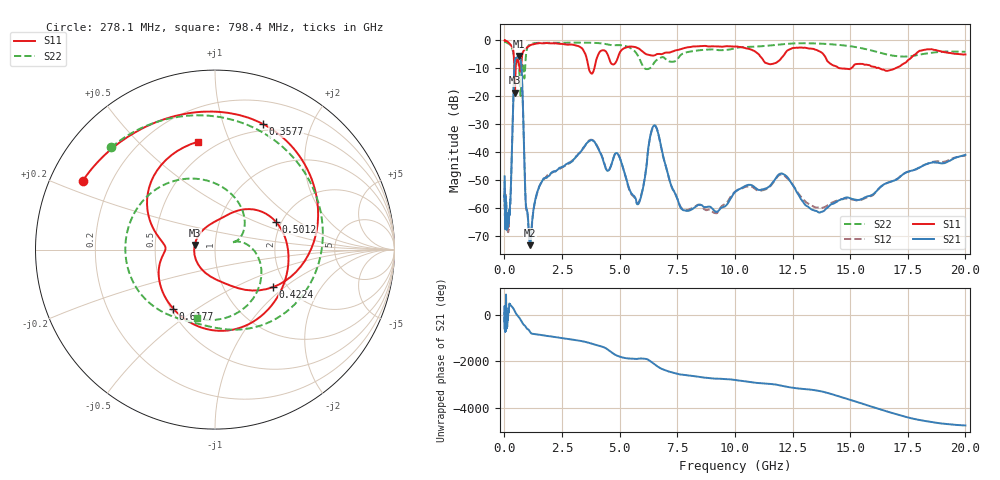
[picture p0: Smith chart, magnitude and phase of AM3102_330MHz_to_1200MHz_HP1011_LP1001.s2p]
! Date/Time: Tue, Sep 11, 2018 5:20 PM
! Network Analyzer: Agilent Technologies E8362B Rev: A.07.50.63
! Sweep from 0.010 to 20.000 GHz, 1601 Points, Sweep Type: LOG
! Power Supply: 4.949 V, 0.001 A
# Hz S DB R 50
!freq MagS11 AngS11 MagS21 AngS21 MagS12 AngS12 MagS22 AngS22
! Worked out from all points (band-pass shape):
!   1601 points, 10 MHz to 20 GHz, reference 50 ohm
!   highest |S21| = -5.53 dB at 638.6 MHz (marker M1); lowest = -73.4 dB at 1.113 GHz (marker M2)
!   |S21| within 3 dB of the highest: 440.3 MHz to 728.7 MHz (288.4 MHz wide, 49.3 % of centre)
!   lowest |S11| = -18.7 dB at 455.8 MHz (marker M3), VSWR 1.26, Z = 39.8 + j2.04 ohm
!   |S11| at or under -10 dB: 3.662 GHz to 3.902 GHz (240.6 MHz wide, 6.36 % of centre); 14.62 GHz to 15.03 GHz (408.4 MHz wide, 2.75 % of centre); 16.29 GHz to 16.95 GHz (666.5 MHz wide, 4.01 % of centre)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
!   |S22| runs from -19.8 to -0.2 dB; largest |S21 - S12| = 0.0096
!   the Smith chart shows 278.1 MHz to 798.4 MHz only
!   S11 on the Smith chart (normalised r, x): 278.1 MHz: 0.10, +0.24; 357.7 MHz: 0.43, +1.36; 422.4 MHz: 1.69, -0.83; 501.2 MHz: 1.87, +0.67; 617.7 MHz: 0.51, -0.40; 798.4 MHz: 0.40, +0.77
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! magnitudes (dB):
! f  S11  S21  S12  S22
! 10 MHz  0.0  -48.6  -50.8  -0.2
! 35.55 MHz  0.0  -64.5  -63.8  -0.4
! 126.4 MHz  -0.4  -64.7  -65.2  -0.9
! 278.1 MHz  -1.6  -53.4  -53.9  -1.8
! 357.7 MHz  -2.5  -29.3  -29.4  -3.4
! 422.4 MHz  -8.3  -11.3  -11.3  -6.1
! 447.2 MHz  -18.1  -7.8  -7.9  -7.3
! 455.8 MHz  -18.7  -7.2  -7.3  -7.5
! 501.2 MHz  -8.6  -6.3  -6.3  -6.3
! 617.7 MHz  -7.9  -5.6  -5.7  -8.4
! 638.6 MHz  -8.8  -5.5  -5.6  -10.2
! 798.4 MHz  -4.3  -21.7  -21.7  -8.1
! 920.7 MHz  -3.0  -57.0  -57.8  -6.8
! 1.113 GHz  -1.7  -73.4  -73.6  -1.4
! 1.59 GHz  -1.0  -51.0  -51.1  -0.8
! 3.775 GHz  -11.8  -35.6  -35.5  -0.8
! 5.652 GHz  -2.3  -55.9  -56.2  -3.8
! 6.518 GHz  -5.3  -30.4  -30.5  -7.7
! 7.92 GHz  -2.5  -61.0  -60.7  -4.2
! 12.03 GHz  -6.2  -47.6  -48.1  -1.4
! 13.74 GHz  -4.2  -61.4  -60.1  -1.1
! 20 GHz  -5.0  -40.9  -41.3  -4.0
